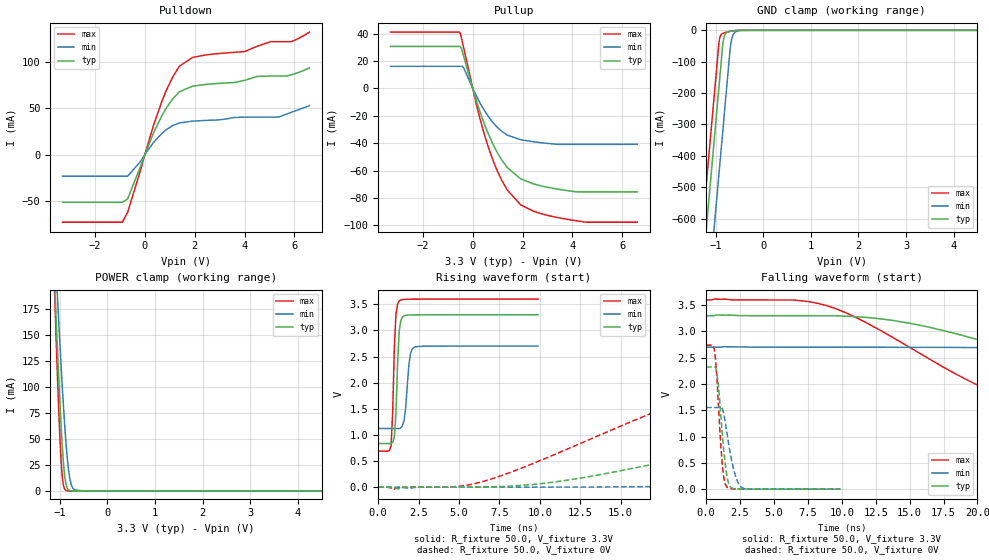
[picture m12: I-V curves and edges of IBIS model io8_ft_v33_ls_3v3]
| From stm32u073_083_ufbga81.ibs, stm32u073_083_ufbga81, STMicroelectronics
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[Model]   io8_ft_v33_ls_3v3
Model_type I/O
Polarity   Non-Inverting
Enable   Active-Low
| CAP_THRESHOLD on pad IOFT is "UDTCAPC" :
| Rising=30.0% of vddiom   Falling=70.0% of vddiom
| C_comp min and max val. don't necessarily correlate with the min and max pvt
| but are the smallest and greatest pad capacitance found.
| var   typ   min   max
C_comp   2.27941pF  2.25177pF  2.68147pF
|C_comp_pullup   1.26014pF  1.27541pF  1.50400pF
|C_comp_pulldown   1.01927pF  976.35715fF  1.17747pF
Vinl = 810.0mV
Vinh = 2.52V
Vmeas = 1.65V   | Reference voltage for timing measurements
Cref  = 50.0pF   | Timing specification test load capacitance value
Rref  = 100.0MOhm   | Timing specification test load resistance value
Vref  = 1.65V   | Timing specification test load voltage
[Model Spec]
| TIME_THRESHOLD on pin ZIV33M is "CMOS" :
| Rising=50.0% of vddiom   Falling=50.0% of vddiom
Vinl 1.34770V 1.11470V 1.44970V
Vinh 1.77530V 1.49030V 1.90330V
| variable   typ   min   max
[Temperature Range] 25.0 140.0 -40.0
| variable   typ   min   max
[Voltage Range] 3.3V 2.7V 3.6V
| variable   typ   min   max
[POWER Clamp Reference] 3.3V 2.7V 3.6V
| variable   typ   min   max
[GND Clamp Reference] 0V 0V 0V
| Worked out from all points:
|   slope of the pulldown table from 0 to 0.495 V, typ, clamps not added: 15.6 ohm
|   slope of the pullup table from 0 to 0.495 V, typ, clamps not added: 18.1 ohm
|   GND clamp passes 1 mA (typ) near -0.60 V on its own axis
|   POWER clamp passes 1 mA (typ) near -0.81 V on its own axis
|   rising waveform, R_fixture 50.0, V_fixture 3.3V: 20-80 % time 190ps typ, 251ps min, 181ps max; typ from 0.835 V to 3.3 V
|   falling waveform, R_fixture 50.0, V_fixture 3.3V: 20-80 % time 21.2ns typ, 46.8ns min, 13.7ns max; typ from 3.3 V to 0.835 V
|   rising waveform, R_fixture 50.0, V_fixture 0V: 20-80 % time 24.1ns typ, 57.5ns min, 14.4ns max; typ from 0 V to 2.33 V
|   falling waveform, R_fixture 50.0, V_fixture 0V: 20-80 % time 472ps typ, 664ps min, 394ps max; typ from 2.33 V to 0 V
[POWER Clamp]
-3.3V     2.991A     2.546A     3.694A
-1.11V    202.2mA    242.3mA    190.9mA
-1.09V    180mA      223.6mA    163.4mA
-1.05V    136.9mA    187mA      110.9mA
-1.01V    96.55mA    151.6mA    64.02mA
-970mV    60.39mA    117.9mA    27.41mA
-930mV    31.08mA    86.54mA    7.282mA
-860mV    4.779mA    40.5mA     315.2uA
-810mV    823.2uA    18.15mA    29.21uA
-750mV    88.98uA    4.952mA    1.667uA
-510mV    11.25nA    8.405uA    48.77pA
6.6V      0A         0A         0A
[GND Clamp]
-3.3V     -4.209A    -4.487A    -4.067A
-1.41V    -996.3mA   -1.274A    -854.3mA
-1.25V    -724.3mA   -1.002A    -582.3mA
-1.21V    -656.3mA   -933.6mA   -514.3mA
-930mV    -180.3mA   -457.6mA   -39.53mA
-900mV    -129.3mA   -406.6mA   -18.05mA
-840mV    -33.79mA   -304.6mA   -9.105mA
-790mV    -10.15mA   -219.6mA   -6.665mA
-680mV    -2.476mA   -41.57mA   -2.768mA
-630mV    -1.406mA   -13.77mA   -1.51mA
-530mV    -268.4uA   -1.762mA   -214.9uA
6.6V      830.6pA    196nA      594.5pA
| variable   typ   min   max
[Pullup Reference] 3.3V 2.7V 3.6V
| variable   typ   min   max
[Pulldown Reference] 0V 0V 0V
[Pullup]
-3.3V     30.64mA    16.16mA    41.13mA
-530mV    30.64mA    16.16mA    41.01mA
-470mV    29.67mA    16.16mA    37.87mA
-370mV    23.8mA     15.16mA    30.04mA
250mV     -14.78mA   -9.185mA   -19.21mA
730mV     -37.54mA   -23mA      -48.39mA
990mV     -46.97mA   -28.45mA   -60.4mA
1.39V     -57.81mA   -34.14mA   -74.25mA
1.92V     -65.96mA   -37.4mA    -84.89mA
2.7V      -70.92mA   -39.51mA   -91.15mA
4.35V     -75.45mA   -40.79mA   -97.1mA
6.6V      -75.45mA   -40.79mA   -97.6mA
[Pulldown]
-3.3V     -51.64mA   -23.39mA   -73.18mA
-900mV    -51.64mA   -23.39mA   -73.04mA
-690mV    -47.97mA   -23.39mA   -62.4mA
350mV     23.63mA    13.27mA    31.99mA
690mV     42.49mA    23.17mA    58.21mA
1.12V     60.48mA    31.51mA    84.25mA
1.39V     68.1mA     34.34mA    95.86mA
1.92V     74.17mA    36.28mA    105.3mA
4V        80.41mA    40.64mA    111.6mA
5.39V     85.07mA    40.9mA     122.4mA
5.88V     86.5mA     45.8mA     122.4mA
6.6V      93.9mA     53mA       132.7mA
[Ramp]
dV/dt_r 1.39485V/24.10412ns 931.92731mV/56.67076ns 1.64323V/14.4182ns
dV/dt_f 1.47908V/21.19607ns 946.45809mV/46.77869ns 1.74613V/13.66639ns
R_load = 50.0
| Removed startup time: 0s 0s 0s  .
| Removed end time: 9.9ns.
[Rising Waveform]
R_fixture   = 50.0
V_fixture   = 3.3V
V_fixture_min = 2.7V
V_fixture_max = 3.6V
0s        834.8mV    1.123V     689.8mV
800ps     833.2mV    1.123V     801mV
900ps     857mV      1.122V     1.461V
1ns       961.9mV    1.122V     2.691V
1.1ns     1.406V     1.121V     3.314V
1.3ns     2.984V     1.119V     3.563V
1.6ns     3.278V     1.274V     3.593V
1.9ns     3.294V     2.344V     3.595V
2.2ns     3.296V     2.671V     3.596V
9.9ns     3.299V     2.7V       3.599V
| Removed startup time: 0s 0s 0s  .
| Removed end time: 499.9ns.
[Falling Waveform]
R_fixture   = 50.0
V_fixture   = 3.3V
V_fixture_min = 2.7V
V_fixture_max = 3.6V
0s        3.3V       2.7V       3.6V
9.5ns     3.299V     2.7V       3.439V
16.4ns    3.084V     2.7V       2.483V
22.7ns    2.642V     2.682V     1.663V
29.1ns    2.135V     2.625V     1.071V
45.2ns    1.191V     2.333V     770.5mV
61.6ns    962.6mV    1.956V     720.6mV
88.4ns    876.5mV    1.45V      697.7mV
131.6ns   843.8mV    1.22V      690.8mV
499.9ns   834.9mV    1.123V     689.8mV
| Removed startup time: 0s 0s 0s  .
| Removed end time: 499.9ns.
[Rising Waveform]
R_fixture   = 50.0
V_fixture   = 0V
V_fixture_min = 0V
V_fixture_max = 0V
0s        -9.486uV   -14.73uV   3.086uV
6.8ns     7.027mV    -113.7uV   135.9mV
18.6ns    543mV      18.88mV    1.614V
25.7ns    1.027V     79.58mV    2.258V
31.1ns    1.365V     153.2mV    2.492V
42.5ns    1.894V     352.7mV    2.652V
56.5ns    2.164V     629.7mV    2.709V
87.9ns    2.293V     1.141V     2.736V
131.6ns   2.322V     1.449V     2.739V
499.9ns   2.325V     1.553V     2.739V
| Removed startup time: 0s 0s 0s  .
| Removed end time: 9.9ns.
[Falling Waveform]
R_fixture   = 50.0
V_fixture   = 0V
V_fixture_min = 0V
V_fixture_max = 0V
0s        2.325V     1.553V     2.739V
600ps     2.332V     1.553V     2.668V
700ps     2.316V     1.553V     2.461V
900ps     1.995V     1.556V     1.634V
1.2ns     1.026V     1.532V     450.5mV
1.5ns     301.6mV    1.13V      52.21mV
1.7ns     80.64mV    800.7mV    14.61mV
2.1ns     7.761mV    308.5mV    3.561mV
2.7ns     2.255mV    21.25mV    2.273mV
9.9ns     383.8uV    232.6uV    549.6uV
